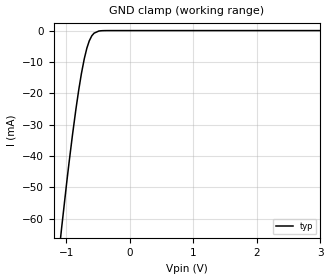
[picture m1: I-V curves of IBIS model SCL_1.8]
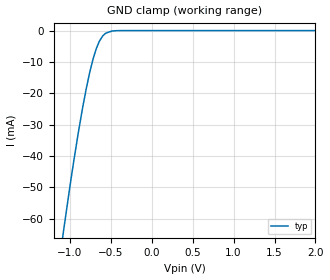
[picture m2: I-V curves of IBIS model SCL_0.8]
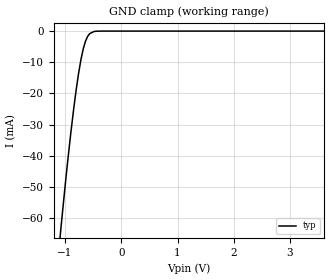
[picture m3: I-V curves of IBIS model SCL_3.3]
|Texas Instruments Incorporated
|tca9848, I2C Switch 8:1X2
[IBIS Ver]   4.1
[File name]   tca9848.ibs
[Date]   09/18/25
[File Rev]   1.0
[Source]
| Texas Instruments Incorporated.
| ASC-INT-MUX
| 12500 TI Blvd
| Dallas, TX - 75243
[Notes]   Revision History:
| Rev 1.0: 09/18/25
| - Initial version of the model
| - Model generated from simulations in SPECTRE
| - C_comp although listed in numerical order of value are
|   obtained from varying PVT conditions. For PVT conditions for
|   each specific value refer the buffer description under
|   respective [Model]. IBIS model user is responsible for using
|   appropriate C_comp to simulate for Signal Integrity.
[Disclaimer]
| This model is designed as an aid for customers of Texas Instruments.
| TI and its licensors and suppliers make no warranties, either expressed
| or implied, with respect to this  model, including the warranties of
| merchantability or fitness for a particular purpose. The model is
| provided solely on an "as is" basis. The entire risk as to its quality
| and performance is with the customer.
| This model is subject to change without notice. Texas Instruments
| Incorporated is not responsible for updating this model.
[Copyright]
(C) Copyright 2025 Texas Instruments Incorporated.All rights reserved.
|  Component TCA9848PW 24-pin - PW package
|  Part # TCA9848PW
[Component]   TCA9848PW
[Manufacturer]  TI
[Package]
|   typ   min   max
R_pkg   0.001   NA   NA
L_pkg   1nH   NA   NA
C_pkg   0.2pF   NA   NA
[Pin]   signal_name   model_name
   1   VDD1   POWER
   2   A0   inbuf
   3   RESET   inbuf
   4   SD0   sterm
   5   SC0   sterm
   6   SD1   sterm
   7   SC1   sterm
   8   SD2   sterm
   9   SC2   sterm
   10   SD3   sterm
   11   SC3   sterm
   12   GND   GND
   13   SD4   sterm
   14   SC4   sterm
   15   SD5   sterm
   16   SC5   sterm
   17   SD6   sterm
   18   SC6   sterm
   19   SD7   sterm
   20   SC7   sterm
   21   A1   inbuf
   22   SCL   SCL
   23   SDA   SDA
   24   VDD2   POWER
[Series Switch Groups]
On 1 /
On 2 /
On 3 /
On 4 /
On 5 /
On 6 /
On 7 /
On 8 /
Off 1 2 3 4 5 6 7 8 /
[Series Pin Mapping]  pin_2 model_name function_table_group
  | 4  23   switch_1.8   1
   5  22   switch_1.8   1
  | 6  23   switch_1.8   2
   7  22   switch_1.8   2
  | 8  23   switch_1.8   3
   9  22   switch_1.8   3
  |10  23   switch_1.8   4
  11  22   switch_1.8   4
  |13  23   switch_1.8   5
  14  22   switch_1.8   5
  |15  23   switch_1.8   6
  16  22   switch_1.8   6
 | 17  23   switch_1.8   7
  18  22   switch_1.8   7
  |19  23   switch_1.8   8
  20  22   switch_1.8   8
|   4  23   switch_0.8   1
|  5  22   switch_0.8   1
|   6  23   switch_0.8   2
|   7  22   switch_0.8   2
|   8  23   switch_0.8   3
|   9  22   switch_0.8   3
|  10  23   switch_0.8   4
|  11  22   switch_0.8   4
|  13  23   switch_0.8   5
|  14  22   switch_0.8   5
|  15  23   switch_0.8   6
|  16  22   switch_0.8   6
|  17  23   switch_0.8   7
|  18  22   switch_0.8   7
|  19  23   switch_0.8   8
|  20  22   switch_0.8   8
|   4  23   switch_3.3   1
|   5  22   switch_3.3   1
|   6  23   switch_3.3   2
|   7  22   switch_3.3   2
|   8  23   switch_3.3   3
|   9  22   switch_3.3   3
|  10  23   switch_3.3   4
|  11  22   switch_3.3   4
|  13  23   switch_3.3   5
|  14  22   switch_3.3   5
|  15  23   switch_3.3   6
|  16  22   switch_3.3   6
|  17  23   switch_3.3   7
|  18  22   switch_3.3   7
|  19  23   switch_3.3   8
|  20  22   switch_3.3   8
[Model Selector] SCL
SCL_1.8 Use for operation at VDD1=1.8V
SCL_0.8 Use for operation at VDD1=0.8V
SCL_3.3 Use for operation at VDD1=3.3V
[Model Selector] SDA
SDA_3.3 Use for operation at VDD1=3.3V
SDA_0.8 Use for Operation at VDD1=0.8V
SDA_1.8 Use for Operation at VDD1=1.8
[Model Selector] sterm
sterm_1.8 Use for operation
sterm_0.8 Use for operation
sterm_3.3 Use for operation
[Model Selector] inbuf
inbuf_1.8 Use for operation at VDD1=1.8V
inbuf_0.8 Use for operation at VDD1=0.8V
inbuf_3.3 Use for operation at VDD1=3.3V
| switch_1.8
[Model]   switch_1.8
Model_type   Series_switch
|   typ   min   max
C_comp   12pF   NA   NA
[Voltage Range]   1.8   NA   NA
[Temperature Range]   27   NA   NA
[On]
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[Off]
|   typ   min   max
[R Series]   10G   NA   NA
| switch_0.8
[Model]   switch_0.8
Model_type   Series_switch
|   typ   min   max
C_comp   12pF   NA   NA
[Voltage Range]   0.8   NA   NA
[Power Clamp Reference]   0.8   NA   NA
[Temperature Range]   27   NA   NA
[On]
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[Off]
|   typ   min   max
[R Series]   10G   NA   NA
| switch_3.3
[Model]   switch_3.3
Model_type   Series_switch
|   typ   min   max
C_comp   12pf   NA   NA
[Voltage Range]   3.3   NA   NA
[Power Clamp Reference]   3.3   NA   NA
[Temperature Range]   27   NA   NA
[On]
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[Off]
|   typ   min   max
[R Series]   10G   NA   NA
| Models and submodels in the file (15): SCL_1.8 (Input), SCL_0.8 (Input), SCL_3.3 (Input), switch_1.8 (Series_switch), switch_0.8 (Series_switch), switch_3.3 (Series_switch), sterm_1.8 (Terminator), sterm_0.8 (Terminator), sterm_3.3 (Terminator), inbuf_1.8 (Input), inbuf_0.8 (Input), inbuf_3.3 (Input), SDA_3.3 (I/O_open_drain), SDA_1.8 (I/O_open_drain), SDA_0.8 (I/O_open_drain)
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| SCL_1.8
[Model]   SCL_1.8
Model_type   Input
Vinl = .54
Vinh = 1.26
|   typ   min   max
C_comp   10pF   NA   NA
[Voltage Range]   1.8   NA   NA
[Temperature Range]   27   NA   NA
[Power Clamp Reference]   1.8   NA   NA
[GND Clamp Reference]   0   NA   NA
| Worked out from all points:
|   GND clamp passes 1 mA (typ) near -0.57 V on its own axis
[GND Clamp]
|   Voltage   I(typ)   I(min)   I(max)
-1.8V     -216.9mA   NA         NA
-1.173V   -82.26mA   NA         NA
-1.073V   -63.03mA   NA         NA
-981.8mV  -46.59mA   NA         NA
-900.6mV  -33.11mA   NA         NA
-846.9mV  -24.95mA   NA         NA
-760.5mV  -13.64mA   NA         NA
-675.5mV  -5.607mA   NA         NA
-638mV    -3.304mA   NA         NA
-562.4mV  -828.1uA   NA         NA
-369.7mV  -5.338uA   NA         NA
3.6V      0A         NA         NA
[POWER Clamp]
|   Voltage   I(typ)   I(min)   I(max)
-1.8V     0A         NA         NA
0V        0A         NA         NA
1.8V      0A         NA         NA
3.6V      0A         NA         NA
6V        0A         NA         NA
| SCL_0.8
[Model]   SCL_0.8
Model_type   Input
Vinl = 0.24
Vinh = .56
|   typ   min   max
C_comp   10pF   NA   NA
[Voltage Range]   0.8   NA   NA
[Temperature Range]   27   NA   NA
[Power Clamp Reference]   0.8   NA   NA
[GND Clamp Reference]   0   NA   NA
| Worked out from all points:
|   GND clamp passes 1 mA (typ) near -0.57 V on its own axis
[GND Clamp]
|   Voltage   I(typ)   I(min)   I(max)
-1.8V     -216.9mA   NA         NA
-1.173V   -82.26mA   NA         NA
-1.073V   -63.03mA   NA         NA
-981.8mV  -46.59mA   NA         NA
-900.6mV  -33.11mA   NA         NA
-846.9mV  -24.95mA   NA         NA
-760.5mV  -13.64mA   NA         NA
-675.5mV  -5.607mA   NA         NA
-638mV    -3.304mA   NA         NA
-562.4mV  -828.1uA   NA         NA
-369.7mV  -5.338uA   NA         NA
3.6V      0A         NA         NA
[POWER Clamp]
|   Voltage   I(typ)   I(min)   I(max)
-1.8V     0A         NA         NA
0V        0A         NA         NA
1.8V      0A         NA         NA
3.6V      0A         NA         NA
6V        0A         NA         NA
| SCL_3.3
[Model]   SCL_3.3
Model_type   Input
Vinl = 1
Vinh = 2.3
|   typ   min   max
C_comp   10pF   NA   NA
[Voltage Range]   3.3   NA   NA
[Temperature Range]   27   NA   NA
[Power Clamp Reference]   3.3   NA   NA
[GND Clamp Reference]   0   NA   NA
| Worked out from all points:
|   GND clamp passes 1 mA (typ) near -0.57 V on its own axis
[GND Clamp]
|   Voltage   I(typ)   I(min)   I(max)
-1.8V     -216.9mA   NA         NA
-1.173V   -82.26mA   NA         NA
-1.073V   -63.03mA   NA         NA
-981.8mV  -46.59mA   NA         NA
-900.6mV  -33.11mA   NA         NA
-846.9mV  -24.95mA   NA         NA
-760.5mV  -13.64mA   NA         NA
-675.5mV  -5.607mA   NA         NA
-638mV    -3.304mA   NA         NA
-562.4mV  -828.1uA   NA         NA
-369.7mV  -5.338uA   NA         NA
3.6V      0A         NA         NA
[POWER Clamp]
|   Voltage   I(typ)   I(min)   I(max)
-1.8V     0A         NA         NA
0V        0A         NA         NA
1.8V      0A         NA         NA
3.6V      0A         NA         NA
6V        0A         NA         NA
